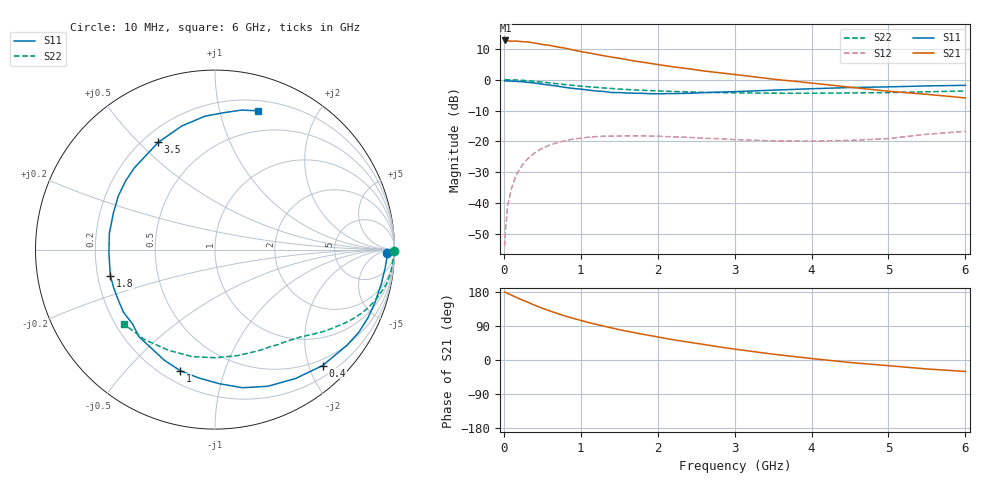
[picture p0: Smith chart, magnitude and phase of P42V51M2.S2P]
! SIEMENS Small Signal Semiconductors
! BFP182
! Si NPN RF Bipolar Junction Transistor in SOT143
! VCE = 2.5 V  IC = 1.2 mA
! Common Emitter S-Parameters:  March  1996
# GHz  S  MA  R  50
!  f  S11  S21  S12  S22
! GHz  MAG  ANG  MAG  ANG  MAG  ANG  MAG  ANG
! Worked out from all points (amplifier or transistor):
!   36 points, 10 MHz to 6 GHz, reference 50 ohm
!   highest |S21| = 12.7 dB at 20 MHz (marker M1)
!   |S21| within 3 dB of that: start of sweep to 886 MHz
!   unconditionally stable (mu >= 1): 2.518 GHz to end of sweep
!   at 250 MHz: K = 0.10, MSG = 19.8 dB, |S12| = -27.4 dB
!   at 1.4 GHz: K = 0.57, MSG = 12.8 dB, |S12| = -18.3 dB
!   at 6 GHz: K = 1.05, MAG = 4.1 dB, |S12| = -16.7 dB
!   S11 on the Smith chart (normalised r, x): 10 MHz: 37, -17; 400 MHz: 0.39, -2.24; 1 GHz: 0.27, -0.72; 1.8 GHz: 0.25, -0.12; 3.5 GHz: 0.26, +0.57; 6 GHz: 0.29, +1.32
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0.01  0.956 -1.2  4.223 179.5  0.002 82.8  0.998 -0.4
0.02  0.9592 -2.5  4.323 178.9  0.0035 89.4  0.9999 -0.9
0.05  0.9537 -6.1  4.272 175.5  0.0092 88.9  0.9966 -2.3
0.1  0.9459 -11.9  4.199 171.0  0.0172 81.7  0.9907 -4.5
0.15  0.9388 -18.3  4.237 166.5  0.0266 78.1  0.9882 -6.9
0.2  0.9329 -24.2  4.18 161.9  0.0347 75.3  0.9819 -9.0
0.3  0.9083 -35.9  4.102 153.6  0.0508 68.3  0.9625 -13.3
0.4  0.8817 -47.1  3.928 144.6  0.0649 61.5  0.939 -17.2
0.6  0.8162 -68.9  3.595 129.4  0.0877 49.5  0.8862 -23.9
0.8  0.7478 -88.1  3.234 115.9  0.1028 39.4  0.8321 -29.4
1  0.7021 -106.0  2.852 104.4  0.1128 31.4  0.7868 -33.8
1.1  0.6782 -114.5  2.725 98.9  0.117 27.8  0.7684 -35.8
1.3  0.6445 -131.0  2.446 89.3  0.1211 21.5  0.7342 -39.3
1.5  0.618 -145.6  2.224 80.1  0.1219 16.6  0.704 -42.6
1.8  0.6009 -165.7  1.924 68.0  0.1224 10.8  0.6736 -47.0
2.2  0.5957 171.1  1.614 53.5  0.1182 5.1  0.6439 -53.3
2.8  0.6285 142.3  1.295 34.6  0.1103 1.1  0.6178 -63.6
3.5  0.6761 117.9  1.02 15.4  0.102 2.3  0.604 -77.7
4  0.7131 105.1  0.882 3.9  0.1009 6.3  0.6026 -89.4
4.5  0.7455 94.3  0.755 -6.6  0.1037 9.7  0.6098 -101.9
5.5  0.7918 79.1  0.579 -23.7  0.1304 16.3  0.6365 -128.0
6  0.8098 72.6  0.506 -30.2  0.1454 14.6  0.6561 -140.8
